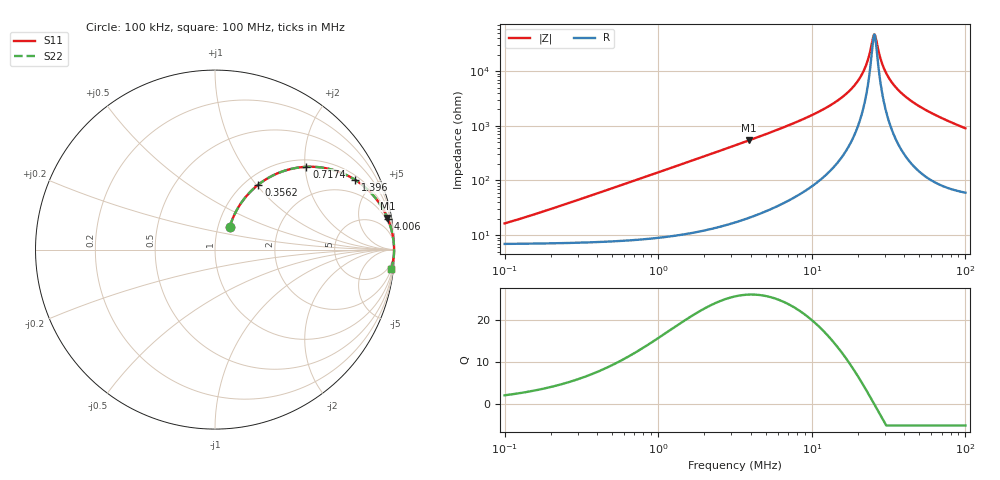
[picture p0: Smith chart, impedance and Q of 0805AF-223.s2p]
# MHz  S  MA  R  50
!Freq  MagS11  AngS11  MagS21  AngS21  MagS12  AngS12  MagS22  AngS22
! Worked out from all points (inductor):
!   801 points, 100 kHz to 100 MHz, reference 50 ohm
!   read as one part in series: L = 23.3 uH near 142.5 kHz
!   highest Q = 26.1 at 3.903 MHz (marker M1), where L = 22.1 uH
!   self-resonance near 25.46 MHz
!   S11 on the Smith chart (normalised r, x): 100 kHz: 1.14, +0.30; 356.2 kHz: 1.15, +1.03; 717.4 kHz: 1.16, +2.03; 1.396 MHz: 1.20, +3.89; 4.006 MHz: 1, +11; 100 MHz: 2, -18
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0.1  0.152 57.1  0.9264 -7.9  0.9264 -7.9  0.152 57.1
0.3183882  0.3991 57.8  0.8564 -23.2  0.8564 -23.2  0.3991 57.8
0.356247  0.4358 56.3  0.8401 -25.6  0.8401 -25.6  0.4358 56.3
0.7174265  0.6868 42.2  0.6737 -43.2  0.6737 -43.2  0.6868 42.2
1.004987  0.7933 34.0  0.5607 -52.3  0.5607 -52.3  0.7933 34.0
1.395693  0.8716 26.5  0.4471 -60.5  0.4471 -60.5  0.8716 26.5
3.172224  0.9669 12.7  0.2204 -75.0  0.2204 -75.0  0.9669 12.7
3.903424  0.9767 10.4  0.1804 -77.4  0.1804 -77.4  0.9767 10.4
4.005954  0.9777 10.1  0.1759 -77.7  0.1759 -77.7  0.9777 10.1
10.01307  0.9948 3.6  0.06356 -83.5  0.06356 -83.5  0.9948 3.6
14.77307  0.9969 2.0  0.03428 -83.8  0.03428 -83.8  0.9969 2.0
19.14578  0.9976 1.0  0.01762 -81.6  0.01762 -81.6  0.9976 1.0
22.17589  0.9978 0.5  0.008788 -75.2  0.008788 -75.2  0.9978 0.5
23.35617  0.9978 0.3  0.005808 -68.0  0.005808 -68.0  0.9978 0.3
24.81278  0.9979 0.1  0.002769 -39.6  0.002769 -39.6  0.9979 0.1
25.46453  0.9979 0.0  0.002137 -5.7  0.002137 -5.7  0.9979 0.0
26.1334  0.9979 -0.1  0.002512 32.2  0.002512 32.2  0.9979 -0.1
28.98924  0.9978 -0.4  0.007887 73.9  0.007887 73.9  0.9978 -0.4
31.88044  0.9978 -0.8  0.01358 80.1  0.01358 80.1  0.9978 -0.8
37.56982  0.9974 -1.4  0.0239 83.2  0.0239 83.2  0.9974 -1.4
47.44399  0.9965 -2.3  0.03982 83.9  0.03982 83.9  0.9965 -2.3
100  0.9867 -6.3  0.1097 79.9  0.1097 79.9  0.9867 -6.3
